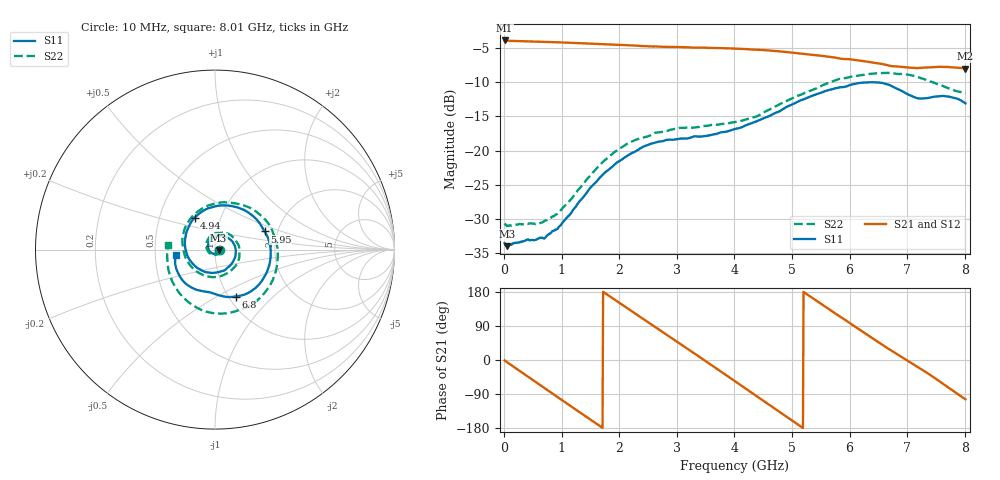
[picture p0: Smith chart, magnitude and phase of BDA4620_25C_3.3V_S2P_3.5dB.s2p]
!Agilent Technologies,E5071B,MY42404982,A.09.10
!Date: Wed May 06 08:56:43 2026
!Data & Calibration Information:
!Freq	S11:SOLT2(ON)	S21:SOLT2(ON)	S12:SOLT2(ON)	S22:SOLT2(ON)
# Hz S RI R 50
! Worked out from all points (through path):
!   801 points, 10 MHz to 8.01 GHz, reference 50 ohm
!   highest |S21| = -3.94 dB at 10 MHz (marker M1); lowest = -8.1 dB at 8.01 GHz (marker M2)
!   group delay of S21, straight-line fit = 286 ps
!   lowest |S11| = -34.0 dB at 60 MHz (marker M3), VSWR 1.04, Z = 52 - j0.242 ohm
!   |S11| at or under -10 dB: start of sweep to end of sweep
!   |S22| runs from -31.0 to -8.7 dB; largest |S21 - S12| = 0.0026
!   S11 on the Smith chart (normalised r, x): 10 MHz: 1.04, -0.00; 4.94 GHz: 0.75, +0.28; 5.95 GHz: 1.71, +0.38; 6.8 GHz: 1.08, -0.61; 8.01 GHz: 0.64, -0.04
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1e7  0.021 -0.00142  0.6349 -0.0136  0.6357 -0.0137  0.0293 -0.00202
6e7  0.0199 -0.00233  0.6284 -0.0727  0.6296 -0.0736  0.0279 -0.00373
3.7e8  0.0166 -0.0145  0.485 -0.3961  0.4854 -0.3974  0.0206 -0.0204
7.3e8  -0.00334 -0.0233  0.139 -0.6038  0.139 -0.6047  -0.00641 -0.0303
1.03e9  -0.0277 -0.0123  -0.1929 -0.5817  -0.1936 -0.5825  -0.0357 -0.0148
1.35e9  -0.039 0.0213  -0.4755 -0.3755  -0.476 -0.376  -0.0487 0.0265
1.64e9  -0.0226 0.0574  -0.5925 -0.0857  -0.5931 -0.0859  -0.0301 0.0701
1.93e9  0.0178 0.0778  -0.5493 0.2187  -0.5497 0.2195  0.0182 0.0963
2.32e9  0.0821 0.0585  -0.2728 0.5132  -0.2738 0.5138  0.0959 0.0738
2.68e9  0.116 -0.00405  0.0863 0.5665  0.0868 0.5669  0.1354 0.00581
3.07e9  0.0907 -0.082  0.4261 0.3757  0.4272 0.3756  0.1188 -0.0855
3.38e9  0.0366 -0.1206  0.5555 0.0937  0.5561 0.0926  0.0571 -0.1372
3.69e9  -0.0331 -0.1281  0.5164 -0.2148  0.5158 -0.216  -0.0305 -0.1511
4.01e9  -0.1069 -0.0955  0.3094 -0.4591  0.3091 -0.46  -0.1207 -0.1073
4.46e9  -0.1673 0.0201  -0.1227 -0.5279  -0.1231 -0.5283  -0.181 0.0338
4.94e9  -0.1142 0.1776  -0.466 -0.2325  -0.4672 -0.2326  -0.0937 0.2139
5.35e9  0.045 0.2469  -0.479 0.1362  -0.4796 0.1366  0.0923 0.2601
5.95e9  0.2758 0.1013  -0.105 0.4528  -0.1049 0.4538  0.3316 0.0708
6.68e9  0.173 -0.2473  0.3643 0.2024  0.3659 0.2025  0.2082 -0.3041
6.8e9  0.1144 -0.2613  0.3904 0.1266  0.3918 0.1265  0.1431 -0.3337
7.36e9  -0.0697 -0.2314  0.3279 -0.2352  0.3284 -0.236  -0.1608 -0.2807
8.01e9  -0.2187 -0.0319  -0.0936 -0.3845  -0.0941 -0.3856  -0.2597 0.0266
